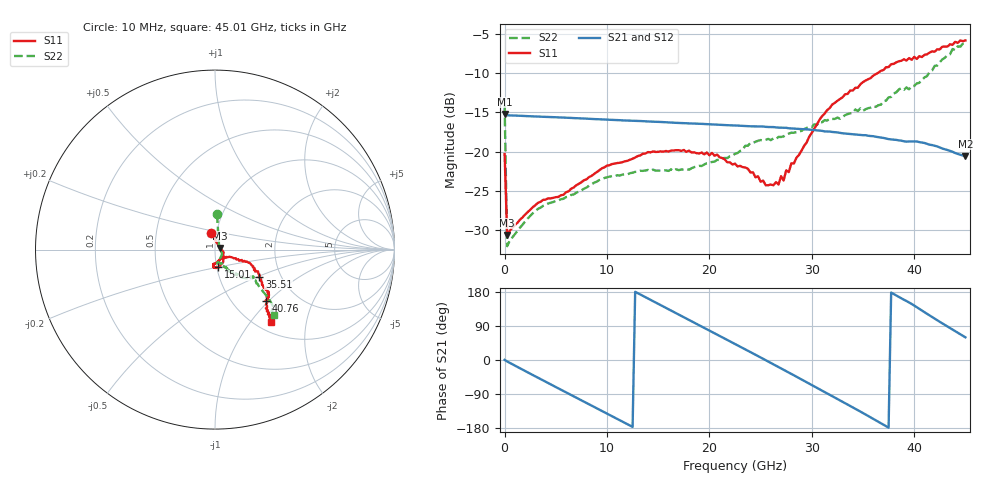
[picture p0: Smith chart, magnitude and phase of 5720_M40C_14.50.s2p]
! Device:  ADRF5720
! Description: 0.5dB LSB GaAs MMIC 6-bit Digital Attenuator
! Frequency:  0.000009 -  40 GHz
! Ports:
!	RF1	= Port 1
!	RF2	= Port 2
! Vdd:  3.3 Volt
! Vss:  -3.3 Volt
! Control:  0/3.3 Volt
! State:  14.50 dB attenuation
! Data:  The device was measured using G-S-G Probes on a matrix board.
!  Data was collected using an calibrated 4 port network analyzer.
!  The reference plane for this measurement is at the launchers.
! Note:  Analog Devices supplies this data as a sample of measured data
!  for this product.  Your particular data for this product may vary.
!  Data was taken at -40 degrees C.
!  Analog Devices reserves the right to change this data at anytime.
# GHZ S DB R 45.0
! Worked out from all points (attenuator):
!   181 points, 10 MHz to 45.01 GHz, reference 45 ohm
!   highest |S21| = -15.19 dB at 10 MHz (marker M1); lowest = -20.6 dB at 45.01 GHz (marker M2)
!   lowest |S11| = -30.6 dB at 260 MHz (marker M3), VSWR 1.06, Z = 47.6 + j0.827 ohm
!   |S11| at or under -10 dB: start of sweep to 36.43 GHz
!   |S22| runs from -32.0 to -6.2 dB; largest |S21 - S12| = 0.00065
!   S11 on the Smith chart (normalised r, x): 10 MHz: 0.94, +0.18; 15.01 GHz: 1.02, -0.20; 35.51 GHz: 1.55, -0.51; 40.76 GHz: 1.41, -0.95; 45.01 GHz: 1.17, -1.27
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0.01  -20.30 104.7  -15.19 0.2  -15.20 0.2  -14.08 86.8
0.26  -30.58 17.1  -15.37 -3.9  -15.38 -3.9  -32.02 18.1
3.26  -26.51 -13.7  -15.53 -46.7  -15.56 -46.7  -27.28 -27.5
5.76  -25.48 -30.4  -15.66 -81.9  -15.69 -81.9  -25.99 -46.8
7.76  -23.63 -44.4  -15.78 -110.0  -15.80 -110.0  -24.71 -61.5
11.51  -21.33 -62.5  -16.01 -162.6  -16.03 -162.6  -22.92 -74.8
15.01  -20.02 -79.3  -16.20 148.2  -16.22 148.1  -22.41 -78.5
15.26  -19.96 -80.6  -16.22 144.6  -16.24 144.6  -22.42 -78.8
19.01  -20.23 -93.2  -16.45 91.8  -16.47 91.7  -21.80 -69.3
20.76  -20.37 -94.4  -16.56 67.0  -16.58 67.0  -21.04 -63.9
22.76  -21.88 -96.5  -16.68 38.7  -16.71 38.6  -20.17 -63.0
23.76  -22.16 -90.0  -16.76 24.6  -16.78 24.5  -19.25 -61.8
25.51  -24.27 -64.8  -16.84 -0.6  -16.86 -0.8  -18.49 -58.3
26.76  -24.17 -45.4  -16.94 -18.6  -16.97 -18.8  -18.12 -56.8
27.01  -23.11 -42.7  -16.95 -22.1  -16.98 -22.3  -18.13 -58.3
30.26  -17.04 -22.2  -17.25 -69.8  -17.27 -69.9  -16.51 -55.8
32.01  -14.00 -21.4  -17.49 -95.6  -17.52 -95.7  -15.84 -52.1
35.51  -10.78 -31.3  -17.97 -147.8  -17.99 -147.9  -14.47 -46.6
37.76  -8.87 -38.5  -18.44 177.9  -18.47 177.7  -13.03 -44.8
40.76  -7.96 -45.3  -18.84 130.8  -18.87 130.6  -10.89 -37.2
43.76  -6.40 -50.0  -20.01 80.1  -20.03 79.9  -6.93 -44.3
45.01  -5.85 -52.1  -20.56 59.8  -20.60 59.7  -6.20 -48.0
